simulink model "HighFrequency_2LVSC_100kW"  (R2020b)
settings: Solver=ode45  StartTime=0.0  StopTime=360  RelTol=1e-4  EnableMultiTasking=on
undefined symbols (not defined in the file): A, A_extheat, A_mp, AceH, AceL, ad0H, ad0L, ad1H, ad1L, ad2H, ad2L, AfH, AfL, at0H, at0L, at1H, at1L, at2H, at2L, C_V_ref, Cha1, CjcD, CjcT, Converters, Cp_Cu, Cp_wall, filter, FILTER_INT, fs, Grid_V, IGBT_len, IGBT_wid, Iq_init, J, k_box, k_mp, k_tp, kI_speed, kP_speed, L_equi, L_f1, Len_mp, Ls, nSpp, omega_m_init, omega_s, p, phi_pm, R1_cauer, R1D_bp, R2_cauer, R_f1, R_jc1, R_jc2, R_jc3, R_jc4, R_wall, Radius, RceH, RceL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
libraries: simulink x5, powerlib_meascontrol x2, pid_lib x2, cstblocks x1
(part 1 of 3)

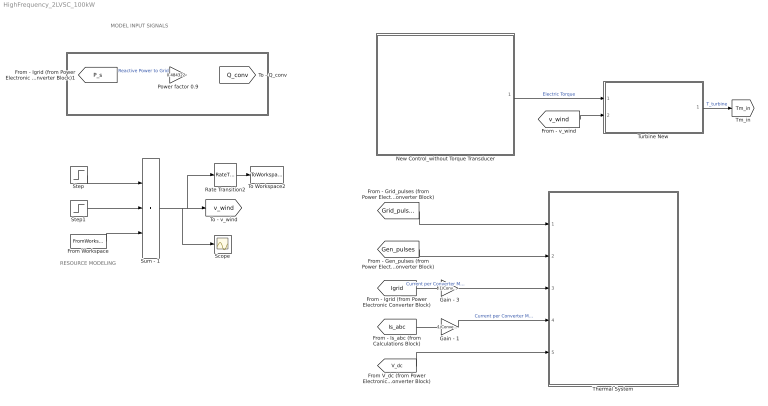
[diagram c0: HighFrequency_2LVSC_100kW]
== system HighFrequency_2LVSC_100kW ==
  note: RESOURCE MODELING
  note: MODEL INPUT SIGNALS
  "    " : Subsystem
  From Workspace : FromWorkspace  VariableName=vel_series  SampleTime=0.25
  Gain - 1 : Gain  Gain=1/Converters
  Gain - 3 : Gain  Gain=-1/Converters
  New Control_without Torque Transducer : Subsystem
  Power factor 0.9 : Gain  Gain=0.484322
  Rate Transition2 : RateTransition  OutPortSampleTime=1
  Scope : Scope
  Step : Step  Time=10  Before=0.52  After=v_tide  SampleTime=0
  Step1 : Step  Time=60  After=-v_tide  SampleTime=0
  Sum - 1 : Sum  Inputs=+++  InputSameDT=on  SaturateOnIntegerOverflow=on
  Thermal System : Subsystem
  To Workspace2 : ToWorkspace  VariableName=v_tide_simulink  SaveFormat=Structure With Time  SampleTime=-1
  Turbine New : Subsystem
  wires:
  New Control_without Torque Transducer/1(Torque_e) -> Turbine New/1(Electric Torque)  "Electric Torque"
  [P_s] -> Power factor 0.9/1  "Reactive Power to Grid"
  [v_wind] -> Turbine New/2(Tide Speed)
  Power factor 0.9/1 -> [Q_conv]
  Turbine New/1(T_load) -> [Tm_in]  "T_turbine"
  Step/1 -> Sum - 1/1
  [Is_abc] -> Gain - 1/1
  [V_dc] -> Thermal System/5(V_dc)
  Gain - 1/1 -> Thermal System/4(I_abc)  "Current per Converter Module"
  [Igrid] -> Gain - 3/1  "Current per Converter Module"
  [Gen_pulses] -> Thermal System/2(Gen_D)
  [Grid_pulses] -> Thermal System/1(Grid_D)
  Gain - 3/1 -> Thermal System/3(Igrid)
  Step1/1 -> Sum - 1/2
  From Workspace/1 -> Sum - 1/3
  Rate Transition2/1 -> To Workspace2/1
  Sum - 1/1 -> Scope/1, Rate Transition2/1, [v_wind]

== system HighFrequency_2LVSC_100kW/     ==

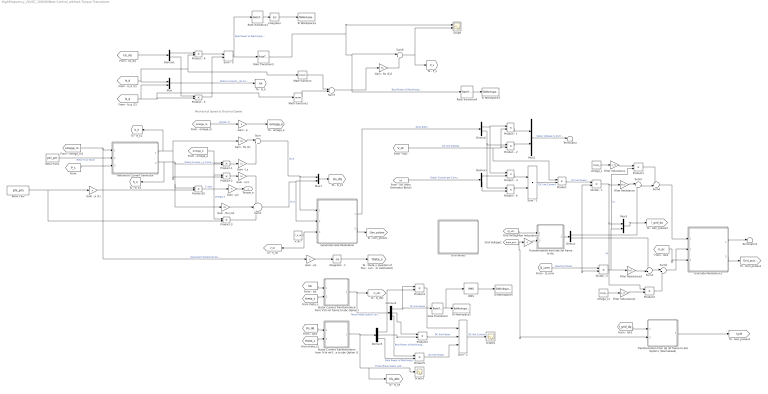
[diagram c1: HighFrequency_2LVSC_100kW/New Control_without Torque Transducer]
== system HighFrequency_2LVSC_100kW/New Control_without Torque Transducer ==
  note: Mechanical Speed to Electrical Speed
  Demux{,1..3} (4 alike) : Demux  Outputs=2
  Demux4 : Demux  Outputs=3
  Demux5 : Demux  Outputs=3
  Divide - 1 : Product  Inputs=*/
  Divide - 2 : Product  Inputs=*/
  Filter Inductance : Gain  Gain=L_f1
  Filter Inductance1 : Gain  Gain=L_f1
  Filter Inductance2 : Gain  Gain=-1
  Filter Resistance : Gain  Gain=R_f1
  "Filter Resistance2 " : Gain  Gain=R_f1
  Gain - Ls : Gain  Gain=Ls
  Gain - Ls1 : Gain  Gain=Ls
  Gain - Rs (1) : Gain  Gain=Rs
  Gain - Rs (1)1 : Gain  Gain=Rs
  Gain - Rs (1)2 : Gain  Gain=Rs
  Gain - p : Gain  Gain=p
  Gain - p (1) : Gain  Gain=p
  Gain - p1 : Gain  Gain=p
  Gain - p2 : Gain
  Generator-Side Modulation : Subsystem
  Grid Values : Subsystem
  Grid-Side Modulation1 : Subsystem
  Integrator : Integrator
  Integrator - 1 : Integrator  InitialCondition=theta_init
  Math Function : Math  Operator=square  SignedPower=on
  Math Function1 : Math  Operator=square  SignedPower=on
  Mux{,1..3} (4 alike) : Mux  Inputs=2
  Product{,1..5} (6 alike) : Product
  Product - {1..3,6} (4 alike) : Product
  Product - 4 : Product  InputSameDT=on  RndMeth=Zero  SaturateOnIntegerOverflow=on
  Product - 5 : Product  InputSameDT=on  RndMeth=Zero  SaturateOnIntegerOverflow=on
  Product-1 : Product  InputSameDT=on  RndMeth=Zero  SaturateOnIntegerOverflow=on
  Product-2 : Product  InputSameDT=on  RndMeth=Zero  SaturateOnIntegerOverflow=on
  Product-3 : Product  InputSameDT=on  RndMeth=Zero  SaturateOnIntegerOverflow=on
  Product10 : Product  InputSameDT=on  RndMeth=Zero  SaturateOnIntegerOverflow=on
  RMS : powerlib_meascontrol/Measurements/RMS  TrueRMS=on  Freq=13.7  RMSInit=120  Ts=0
  Rate Transition1 : RateTransition  OutPortSampleTime=0.001
  Rate Transition2 : RateTransition  OutPortSampleTime=0.001
  Rate Transition3 : RateTransition  OutPortSampleTime=0.1
  Rate Transition4 : RateTransition  OutPortSampleTime=1
  Reference Current Generator : Subsystem
  Rotor Flux : Constant  Value=phi_pm
  Rotor Flux1 : Constant  Value=phi_pm
  Scope : Scope  NumInputPorts=2
  Scope1 : Scope
  Scope2 : Scope
  Stator Current Transformation from 'k'th ref frame to abc Option I : Subsystem
  Stator Current Transformation from 'k'th ref frame to abc Option I1 : Subsystem
  Sum : Sum  Inputs=|+-
  Sum - 1 : Sum
  Sum - 2 : Sum  Inputs=+++
  Sum - 3 : Sum  InputSameDT=on  SaturateOnIntegerOverflow=on
  Sum1 : Sum  Inputs=+|+|+
  Sum2 : Sum  Inputs=|++
  Sum3 : Sum  Inputs=++|
  Sum4 : Sum  Inputs=-+|
  Sum5 : Sum  Inputs=|++
  Sum6 : Sum  Inputs=|+-
  Sum7 : Sum  Inputs=|++
  Terminator : Terminator
  Terminator1 : Terminator
  To Workspace1 : ToWorkspace  VariableName=P_gen  SaveFormat=Structure With Time  SampleTime=-1
  To Workspace2 : ToWorkspace  VariableName=IsGen_a  SaveFormat=Structure With Time  SampleTime=-1
  To Workspace3 : ToWorkspace  VariableName=Power_Gen1  SaveFormat=Structure With Time  SampleTime=1
  To Workspace4 : ToWorkspace  VariableName=IsGen_arms  SaveFormat=Structure With Time  SampleTime=-1
  "Transformation from abc ref frame to dq " : Subsystem
  Transformation from dq ref frame to abc Option I (Normalised) : Subsystem
  V_dc* : Constant  Value=C_V_ref
  omega_s : Constant  Value=omega_s
  omega_s1 : Constant  Value=omega_s
  Torque_e : Outport  VectorParamsAs1DForOutWhenUnconnected=off
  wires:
  [omega_m] -> Gain - p/1  "omega_m"
  Gain - p/1 -> [omega_e]
  Rotor Flux/1 -> Product-3/2, Gain - p (1)/1
  Gain - p (1)/1 -> Product10/2
  Product10/1 -> Gain - p2/1  "T_elec"
  Mux/1 -> [Isk]  "Stator Currents - dq Components"
  Demux1/1 -> Product - 4/1
  Demux1/2 -> Product - 5/1
  Product - 4/1 -> Sum - 3/1
  Product - 5/1 -> Sum - 3/2
  Sum - 3/1 -> Rate Transition1/1, Rate Transition3/1  "Real Power of Machine(pu)"
  [Is_d] -> Product - 4/2, Math Function/1, Mux/1
  [Is_q] -> Mux/2, Math Function1/1, Product - 5/2
  [Us_dq] -> Demux1/1
  Rotor Flux1/1 -> Reference Current Generator/2(Rotor Flux)  "Rotor Flux Value"
  [omega_m] -> Gain - p1/1, Reference Current Generator/1(omega_m)  "Generator Rotational Speed"
  Product-1/1 -> Gain - Ls/1
  [omega_e] -> Product-3/1, Product-2/1, Product-1/1  "omega_e"
  Reference Current Generator/2(I_q ref) -> [Is_q], Product-1/2, Gain - Rs (1)1/1, Product10/1  "Stator Current - q Component"
  Gain - Rs (1)/1 -> Sum/1
  Gain - Ls/1 -> Sum/2
  Sum/1 -> Generator-Side Modulation/1(Vd), Mux1/1  "Us_d"
  Reference Current Generator/1(I_d ref) -> [Is_d], Product-2/2, Gain - Rs (1)/1
  Product-2/1 -> Gain - Ls1/1
  Gain - Rs (1)1/1 -> Sum1/2
  Gain - Ls1/1 -> Sum1/1
  Product-3/1 -> Sum1/3
  Sum1/1 -> Generator-Side Modulation/2(Vq), Mux1/2  "Us_q"
  Mux1/1 -> [Us_dq]
  V_dc*/1 -> [V_dc], Generator-Side Modulation/3(Vdc)
  Generator-Side Modulation/2(Dabc) -> [Gen_pulses]
  Gain - p1/1 -> Integrator - 1/1
  Integrator - 1/1 -> [theta_s]
  [Isk] -> Stator Current Transformation from 'k'th ref frame to abc Option I/1("Is_{k}")
  [theta_s] -> Stator Current Transformation from 'k'th ref frame to abc Option I/2(theta_(s))
  Generator-Side Modulation/1(Ddq) -> Demux2/1  "Duty Ratio"
  Demux2/1 -> Product - 3/1, Product - 1/1
  [V_dc] -> Product/1, Product - 2/2, Product - 1/2  "DC link Voltage"
  Product - 1/1 -> Mux2/1
  Product - 2/1 -> Mux2/2
  Mux2/1 -> Terminator/1  "Stator Voltage in dq frame"
  Demux2/2 -> Product - 6/1, Product - 2/1
  [Isk] -> Demux3/1  "Stator Current per Converter Module"
  Demux3/1 -> Product - 3/2
  Demux3/2 -> Product - 6/2
  Product - 3/1 -> Sum - 1/1
  Product - 6/1 -> Sum - 1/2
  Sum - 1/1 -> Product/2  "DC link Current"
  Product/1 -> Divide - 1/1  "DC-link Power"
  [Vg_abc] -> "Transformation from abc ref frame to dq "/1(D_abc)
  [theta_grid] -> Transformation from dq ref frame to abc Option I (Normalised)/2(theta), Filter Inductance2/1
  "Transformation from abc ref frame to dq "/1(D_dq) -> Demux/1
  Demux/1 -> Sum2/2, Divide - 1/2, Divide - 2/2
  Divide - 1/1 -> Mux3/1, Product2/1, Filter Resistance/1  "Id"
  [Q_conv] -> Divide - 2/1  "Reactive Power"
  Divide - 2/1 -> "Filter Resistance2 "/1, Mux3/2, Product1/2  "Iq"
  omega_s/1 -> Filter Inductance/1
  Filter Resistance/1 -> Sum2/1
  "Filter Resistance2 "/1 -> Sum3/2
  Demux/2 -> Sum3/1
  Sum2/1 -> Sum4/2
  Filter Inductance/1 -> Product1/1
  Product1/1 -> Sum4/1
  omega_s1/1 -> Filter Inductance1/1
  Filter Inductance1/1 -> Product2/2
  Sum3/1 -> Sum5/1
  Product2/1 -> Sum5/2
  Sum4/1 -> Grid-Side Modulation1/1(Vd)
  Sum5/1 -> Grid-Side Modulation1/2(Vq)
  [V_dc] -> Grid-Side Modulation1/3(Vdc)
  Grid-Side Modulation1/2(Dabc) -> [Grid_pulses]
  Grid-Side Modulation1/1(Ddq) -> Terminator1/1
  Mux3/1 -> [I_grid_dq]
  [I_grid_dq] -> Transformation from dq ref frame to abc Option I (Normalised)/1(D_dq)
  Transformation from dq ref frame to abc Option I (Normalised)/1(D_abc) -> [Igrid]
  Filter Inductance2/1 -> "Transformation from abc ref frame to dq "/2(theta_(s))
  [Us_dq] -> Stator Current Transformation from 'k'th ref frame to abc Option I1/1("Is_{k}")
  [theta_s] -> Stator Current Transformation from 'k'th ref frame to abc Option I1/2(theta_(s))
  Rate Transition1/1 -> Integrator/1
  Integrator/1 -> To Workspace1/1
  [P_s] -> Reference Current Generator/3("P_in ")
  Gain - p2/1 -> Torque_e/1
  Demux4/2 -> Product3/1
  Demux4/1 -> Product4/1, Rate Transition2/1
  Stator Current Transformation from 'k'th ref frame to abc Option I/1("Is_{abc}") -> Demux4/1, [Is_abc]  "Three Phase Stator Currents"
  Stator Current Transformation from 'k'th ref frame to abc Option I1/1("Is_{abc}") -> [Us_abc], Scope1/1, Demux5/1  "Three Phase Stator voltage"
  Demux5/2 -> Product3/2
  Demux5/1 -> Product4/2
  Demux4/3 -> Product5/1  "Real Power of Machine(pu)"
  Demux5/3 -> Product5/2  "Real Power of Machine(pu)"
  Product3/1 -> Sum - 2/2  "DC-link Power"
  Product4/1 -> Sum - 2/1  "DC-link Power"
  Product5/1 -> Sum - 2/3  "DC-link Power"
  Sum - 2/1 -> Scope2/1  "DC link Current"
  Gain - Rs (1)2/1 -> Sum6/2
  Math Function/1 -> Sum7/1
  Math Function1/1 -> Sum7/2
  Sum7/1 -> Gain - Rs (1)2/1
  Sum6/1 -> [P_s], Scope/2
  RMS/1 -> To Workspace4/1
  Rate Transition2/1 -> RMS/1, To Workspace2/1
  Rate Transition4/1 -> To Workspace3/1
  Rate Transition3/1 -> Rate Transition4/1, Sum6/1, Scope/1  "Real Power of Machine(pu)"

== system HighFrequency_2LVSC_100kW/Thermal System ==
  Grid_D : Inport
  Gen_D : Inport  Port=2
  Igrid : Inport  Port=3
  I_abc : Inport  Port=4
  V_dc : Inport  Port=5
  Select Leg (Select Converter Leg for Thermal Model) : Constant
  Thermal Model - Generator Side : Subsystem
  Thermal Model - Grid Side : Subsystem  Commented=on
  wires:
  Igrid/1 -> Thermal Model - Grid Side/2(I_abc)
  Grid_D/1 -> Thermal Model - Grid Side/1(D_abc)
  V_dc/1 -> Thermal Model - Grid Side/3(V_dc), Thermal Model - Generator Side/3(V_dc)
  I_abc/1 -> Thermal Model - Generator Side/2(I_abc)
  Gen_D/1 -> Thermal Model - Generator Side/1(D_abc)
  Select Leg (Select Converter Leg for Thermal Model)/1 -> [Phase]

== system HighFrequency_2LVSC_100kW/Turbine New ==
  Electric Torque : Inport
  Tide Speed : Inport  Port=2
  Mechanical System : Subsystem
  Product - 1 : Product  Commented=on  RndMeth=Zero
  Rate Transition1 : RateTransition  OutPortSampleTime=Ts_out/5
  Rate Transition2 : RateTransition  OutPortSampleTime=Ts_out/5
  Rotor Model : Subsystem
  Scope : Scope
  To Workspace1 : ToWorkspace  VariableName=Gen_loadT  SaveFormat=Structure With Time  SampleTime=-1
  To Workspace2 : ToWorkspace  VariableName=v_tide_struct  SaveFormat=Structure With Time  SampleTime=-1
  T_load : Outport  VectorParamsAs1DForOutWhenUnconnected=off
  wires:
  Mechanical System/1(omega_m) -> Rotor Model/1(omega_m), Product - 1/2, [omega_m]  "Generator Rotational Speed"
  Electric Torque/1 -> Mechanical System/1(Electric Torque)  "T_elec"
  Rate Transition1/1 -> To Workspace1/1
  Tide Speed/1 -> Rate Transition2/1, Rotor Model/2(Wind Speed)
  Rate Transition2/1 -> To Workspace2/1
  Rotor Model/1(T_load) -> Product - 1/1, Rate Transition1/1, T_load/1, Mechanical System/2(Load Torque)
  Product - 1/1 -> Scope/1

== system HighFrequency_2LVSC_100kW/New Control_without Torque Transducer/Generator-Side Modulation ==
  Vd : Inport
  Vq : Inport  Port=2
  Vdc : Inport  Port=3
  Divide - 1 : Product  Inputs=*/
  Duty Limits : Saturate
  Gain - 1 : Gain  Gain=2
  Mux2 : Mux  Inputs=2
  Third Harmonic Injection : Subsystem
  Transformation from abc ref frame to dq Option I (Normalised) : Subsystem
  Transformation from dq ref frame to abc Option I (Normalised) : Subsystem
  Ddq : Outport  VectorParamsAs1DForOutWhenUnconnected=off
  Dabc : Outport  Port=2  VectorParamsAs1DForOutWhenUnconnected=off
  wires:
  Third Harmonic Injection/1(V_out) -> Duty Limits/1
  Duty Limits/1 -> Gain - 1/1, Transformation from abc ref frame to dq Option I (Normalised)/1(D_abc)
  Gain - 1/1 -> Dabc/1
  Divide - 1/1 -> Transformation from dq ref frame to abc Option I (Normalised)/1(D_dq)  "Duty Ratio"
  Transformation from abc ref frame to dq Option I (Normalised)/1(D_dq) -> Ddq/1
  [theta_s] -> Transformation from dq ref frame to abc Option I (Normalised)/2(theta), Transformation from abc ref frame to dq Option I (Normalised)/2(theta_(s))
  Vdc/1 -> Divide - 1/2
  Mux2/1 -> Divide - 1/1
  Vd/1 -> Mux2/1
  Vq/1 -> Mux2/2
  Transformation from dq ref frame to abc Option I (Normalised)/1(D_abc) -> Third Harmonic Injection/1(V_in)

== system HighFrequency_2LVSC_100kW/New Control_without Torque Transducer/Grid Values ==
  Create 3 Phase Voltage Signal (in lieu of Grid Model) : Subsystem
  Grid Voltage (from Initialisation file) : Constant  Value=Grid_V
  Mux3 : Mux  Inputs=3
  Voltage Angle in dq : Subsystem
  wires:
  Mux3/1 -> Voltage Angle in dq/1(Three Phase Voltages), [Vg_abc], [Usabc]
  Create 3 Phase Voltage Signal (in lieu of Grid Model)/3(Phase C Voltage) -> Mux3/3
  Create 3 Phase Voltage Signal (in lieu of Grid Model)/1(Phase A Voltage) -> Mux3/1
  Grid Voltage (from Initialisation file)/1 -> Create 3 Phase Voltage Signal (in lieu of Grid Model)/1(Grid Voltage)
  Create 3 Phase Voltage Signal (in lieu of Grid Model)/2(Phase B Voltage) -> Mux3/2
  Voltage Angle in dq/1(angle) -> [theta_grid]

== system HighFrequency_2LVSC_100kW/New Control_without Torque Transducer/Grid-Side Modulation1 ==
  Vd : Inport
  Vq : Inport  Port=2
  Vdc : Inport  Port=3
  Divide - 1 : Product  Inputs=*/
  Duty Limits : Saturate
  Gain - 1 : Gain  Gain=2
  Mux2 : Mux  Inputs=2
  Third Harmonic Injection : Subsystem
  Transformation from abc ref frame to dq Option I (Normalised) : Subsystem
  Transformation from dq ref frame to abc Option I (Normalised) : Subsystem
  Ddq : Outport  VectorParamsAs1DForOutWhenUnconnected=off
  Dabc : Outport  Port=2  VectorParamsAs1DForOutWhenUnconnected=off
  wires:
  Third Harmonic Injection/1(V_out) -> Duty Limits/1
  Duty Limits/1 -> Gain - 1/1, Transformation from abc ref frame to dq Option I (Normalised)/1(D_abc)
  Gain - 1/1 -> Dabc/1
  Divide - 1/1 -> Transformation from dq ref frame to abc Option I (Normalised)/1(D_dq)  "Duty Ratio"
  Transformation from abc ref frame to dq Option I (Normalised)/1(D_dq) -> Ddq/1
  [theta_grid] -> Transformation from dq ref frame to abc Option I (Normalised)/2(theta), Transformation from abc ref frame to dq Option I (Normalised)/2(theta_(s))
  Vdc/1 -> Divide - 1/2
  Mux2/1 -> Divide - 1/1
  Vd/1 -> Mux2/1
  Vq/1 -> Mux2/2
  Transformation from dq ref frame to abc Option I (Normalised)/1(D_abc) -> Third Harmonic Injection/1(V_in)

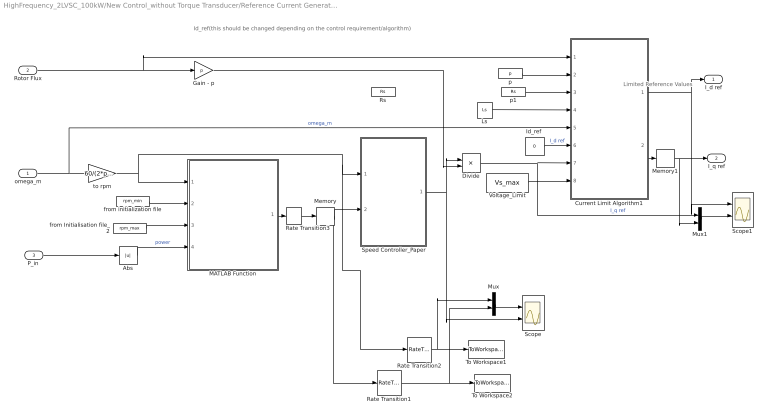
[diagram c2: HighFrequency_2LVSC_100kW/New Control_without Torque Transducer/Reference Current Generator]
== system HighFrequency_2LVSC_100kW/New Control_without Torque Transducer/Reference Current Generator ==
  note: Id_ref(this should be changed depending on the control requirement/algorithm)
  note: Limited Reference Values
  omega_m : Inport
  Rotor Flux : Inport  Port=2
  "P_in " : Inport  Port=3
  Abs : Abs  ZeroCross=off
  Current Limit Algorithm1 : MATLAB Function  TreatAsAtomicUnit=on
  Divide : Product  Inputs=*/
  Gain - p : Gain  Gain=p
  "Id_ref " : Constant  Value=0
  Ls : Constant  Value=Ls
  MATLAB Function : MATLAB Function  TreatAsAtomicUnit=on
  Memory : Memory  InitialCondition=omega_m_init*60/2/pi  InheritSampleTime=on
  Memory1 : Memory  InitialCondition=Iq_init  InheritSampleTime=on
  Mux : Mux  Inputs=2
  Mux1 : Mux  Inputs=2
  Rate Transition1 : RateTransition  OutPortSampleTime=1
  Rate Transition2 : RateTransition  OutPortSampleTime=1
  Rate Transition3 : RateTransition  OutPortSampleTime=0.1
  Rs : Constant  Commented=on  Value=Rs
  Scope : Scope  NumInputPorts=2
  Scope1 : Scope  NumInputPorts=2
  Speed Controller_Paper : Subsystem  mask(Speed controller){SwK=Speed regulation, fn=rpm_rated*p/60, ramp=[-1,1]*2, kp=kP_speed, ki=kI_speed, kd=0, fc=100*100, ctrl_sat=[-1000, 1000]*8.7*1.5*50, p=p, nf=phi_pm, Tsc=1e-5}
      mask prompts: SwK "Regulation type"; fn "Machine nominal frequency (Hz)"; ramp "Speed reference ramp  (rpm/s) [deceleration,acceleration]"; kp "Proportional Gain"; ki "Integral Gain"; kd "Derivative Gain"; fc "Speed measurement - low-pass filter cutoff frequency (Hz)"; ctrl_sat "Controller output torque saturation (N.m) [negative,positive]"; p "Motor pairs of poles"; nf "Machine nominal flux (Wb)"; Tsc "Controller sampling time (s)"
      mask help: This block implements a PI speed regulator.
      mask init:
      | bs=2*30*fn/p;
      | [X1,X1m,X2,X2m,X3,X4,Y1,Y1m,Y2,Y2m,Y3,Y4,color1,color2]=spsdrivelogo;
      | if SwK == 1
      |     set_param(gcb,'MaskVisibilities',{'on','on','on','on','on','on','on','on','on','on','on'})
      | else
      |     set_param(gcb,'MaskVisibilities',{'on','on','off','off','off','off','off','on','on','on','on'})
      | end
  To Workspace1 : ToWorkspace  VariableName=N_gen_plot  SaveFormat=Structure With Time  SampleTime=1
  To Workspace2 : ToWorkspace  VariableName=N_gen_ref  SaveFormat=Structure With Time  SampleTime=1
  Voltage_Limit : Constant  Value=Vs_max
  from Initialisation file_2 : Constant  Value=rpm_max
  from initialization file : Constant  Value=rpm_min
  p : Constant  Value=p
  p1 : Constant  Value=Rs
  to rpm : Gain  Gain=60/(2*pi)
  I_d ref : Outport  VectorParamsAs1DForOutWhenUnconnected=off
  I_q ref : Outport  Port=2  VectorParamsAs1DForOutWhenUnconnected=off
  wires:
  omega_m/1 -> Current Limit Algorithm1/5(omega_m), to rpm/1  "omega_m"
  Rotor Flux/1 -> Current Limit Algorithm1/1(rot_f), Gain - p/1
  "P_in "/1 -> Abs/1
  Current Limit Algorithm1/1(isdref) -> Scope1/1, I_d ref/1
  "Id_ref "/1 -> Current Limit Algorithm1/6(isd)  "I_d ref"
  Current Limit Algorithm1/2(isqref) -> Memory1/1
  Divide/1 -> Mux1/1, Current Limit Algorithm1/7(isq)  "I_q ref"
  Memory1/1 -> Mux1/2, I_q ref/1
  Mux/1 -> Scope/1
  Speed Controller_Paper/1(Torque*) -> Divide/1, Scope/2
  Gain - p/1 -> Divide/2
  from initialization file/1 -> MATLAB Function/2(Nrpmmin)
  from Initialisation file_2/1 -> MATLAB Function/3(Nrpmmax)
  to rpm/1 -> MATLAB Function/1(Nrpm), Speed Controller_Paper/1(N), Rate Transition2/1
  Memory/1 -> Rate Transition1/1, Speed Controller_Paper/2(N*)
  Rate Transition2/1 -> Mux/1, To Workspace1/1
  Rate Transition1/1 -> Mux/2, To Workspace2/1
  Abs/1 -> MATLAB Function/4(P_in)  "power"
  Rate Transition3/1 -> Memory/1
  MATLAB Function/1(N_ref) -> Rate Transition3/1
  Voltage_Limit/1 -> Current Limit Algorithm1/8(Vs_max)
  Ls/1 -> Current Limit Algorithm1/4(Ls)
  p/1 -> Current Limit Algorithm1/2(p)
  p1/1 -> Current Limit Algorithm1/3(Rs)
  Mux1/1 -> Scope1/2

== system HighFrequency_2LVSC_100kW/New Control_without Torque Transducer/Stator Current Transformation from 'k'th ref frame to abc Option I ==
  "Is_{k}" : Inport
  theta_(s) : Inport  Port=2
  Clarke Transform : Subsystem
  Demux : Demux  Outputs=2
  Gain : Gain  Gain=-1
  Mux : Mux  Inputs=3
  "Park Transform " : Subsystem
  "Is_{abc}" : Outport  VectorParamsAs1DForOutWhenUnconnected=off
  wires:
  Clarke Transform/1(out_1) -> Mux/1
  Clarke Transform/3(out_3) -> Mux/3
  Clarke Transform/2(out_2) -> Mux/2
  "Park Transform "/2(out_2) -> Clarke Transform/2(in_2)
  "Park Transform "/1(out_1) -> Clarke Transform/1(in_1)
  Gain/1 -> "Park Transform "/3(in_3)
  "Is_{k}"/1 -> Demux/1
  Mux/1 -> "Is_{abc}"/1
  Demux/1 -> "Park Transform "/1(in_1)
  Demux/2 -> "Park Transform "/2(in_2)
  theta_(s)/1 -> Gain/1

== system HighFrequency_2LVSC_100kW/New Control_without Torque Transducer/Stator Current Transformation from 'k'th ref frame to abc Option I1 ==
  "Is_{k}" : Inport
  theta_(s) : Inport  Port=2
  Clarke Transform : Subsystem
  Demux : Demux  Outputs=2
  Gain : Gain  Gain=-1
  Mux : Mux  Inputs=3
  "Park Transform " : Subsystem
  "Is_{abc}" : Outport  VectorParamsAs1DForOutWhenUnconnected=off
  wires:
  theta_(s)/1 -> Gain/1
  Demux/2 -> "Park Transform "/2(in_2)
  Demux/1 -> "Park Transform "/1(in_1)
  Mux/1 -> "Is_{abc}"/1
  "Is_{k}"/1 -> Demux/1
  Gain/1 -> "Park Transform "/3(in_3)
  "Park Transform "/1(out_1) -> Clarke Transform/1(in_1)
  "Park Transform "/2(out_2) -> Clarke Transform/2(in_2)
  Clarke Transform/2(out_2) -> Mux/2
  Clarke Transform/3(out_3) -> Mux/3
  Clarke Transform/1(out_1) -> Mux/1

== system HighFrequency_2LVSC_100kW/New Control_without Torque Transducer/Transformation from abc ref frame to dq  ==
  D_abc : Inport
  theta_(s) : Inport  Port=2
  Clarke Transform : Subsystem
  Demux : Demux  Outputs=3
  Mux1 : Mux  Inputs=2
  Parks Transform : Subsystem
  D_dq : Outport  VectorParamsAs1DForOutWhenUnconnected=off
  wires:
  Parks Transform/1(out_1) -> Mux1/1
  Parks Transform/2(out_2) -> Mux1/2
  D_abc/1 -> Demux/1
  Mux1/1 -> D_dq/1
  Demux/1 -> Clarke Transform/1(in_1)
  Demux/2 -> Clarke Transform/2(in_2)
  Demux/3 -> Clarke Transform/3(in_3)
  Clarke Transform/1(out_1) -> Parks Transform/1(in_1)
  Clarke Transform/2(out_2) -> Parks Transform/2(in_2)
  theta_(s)/1 -> Parks Transform/3(in_3)

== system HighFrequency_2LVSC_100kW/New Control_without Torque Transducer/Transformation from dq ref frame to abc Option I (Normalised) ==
  D_dq : Inport
  theta : Inport  Port=2
  Clarke Transform : Subsystem
  Demux : Demux  Outputs=2
  Gain : Gain  Gain=-1
  Mux1 : Mux  Inputs=3
  Parks Transform : Subsystem
  D_abc : Outport  VectorParamsAs1DForOutWhenUnconnected=off
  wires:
  Parks Transform/2(out_2) -> Clarke Transform/2(in_2)
  Parks Transform/1(out_1) -> Clarke Transform/1(in_1)
  Gain/1 -> Parks Transform/3(in_3)
  D_dq/1 -> Demux/1
  Mux1/1 -> D_abc/1
  Demux/1 -> Parks Transform/1(in_1)
  Demux/2 -> Parks Transform/2(in_2)
  theta/1 -> Gain/1
  Clarke Transform/3(out_3) -> Mux1/3
  Clarke Transform/2(out_2) -> Mux1/2
  Clarke Transform/1(out_1) -> Mux1/1

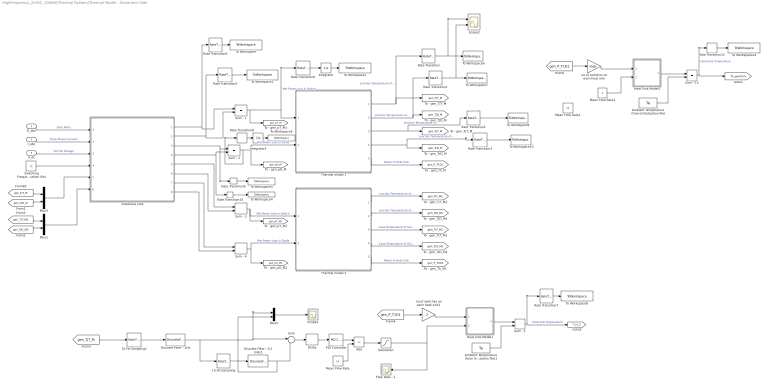
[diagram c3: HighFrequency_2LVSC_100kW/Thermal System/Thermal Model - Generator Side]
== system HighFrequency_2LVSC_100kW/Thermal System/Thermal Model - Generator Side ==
  D_abc : Inport
  I_abc : Inport  Port=2
  V_dc : Inport  Port=3
  10 Hz Sampling : RateTransition  Commented=on  InitialCondition=60  OutPortSampleTime=1e-1
  10 Hz Sampling1 : RateTransition  Commented=on  InitialCondition=60  OutPortSampleTime=1e-3
  Add : Sum  Commented=on  Inputs=-+
  Ambient Temperature (from Initialisation file) : Constant  Value=Ta
  Ambient Temperature (from Initialisation file)1 : Constant  Commented=on  Value=Ta
  Delay : Delay  Commented=on  DelayLength=1  InitialCondition=0  SampleTime=1e-3
  Discrete Filter - 0.1 mHz1 : DiscreteFilter  Commented=on  Numerator=[1 1]  Denominator=[1]  InitialStates=1
  Discrete Filter - 1Hz : DiscreteFilter  Commented=on  Numerator=[1 1]  Denominator=FILTER_INT  InitialStates=filter
  Flow Rate - 1 : Scope
  Heat Sink Model1 : Subsystem  Commented=on
  Heat Sink Model2 : Subsystem
  Instanous Loss : Subsystem
  Integrator : Integrator
  Integrator1 : Integrator
  Mean Flow Rate : Constant  Commented=on  Value=15
  Mean Flow Rate1 : Constant  Commented=on  Value=15
  Mean Flow Rate2 : Constant
  Mux1 : Mux  Inputs=2
  Mux2 : Mux  Commented=on  Inputs=2
  Mux3 : Mux  Inputs=2
  PID Controller : pid_lib/PID Controller  Commented=on  Controller=P  Form=Parallel  TimeDomain=Continuous-time  UseExternalTs=off  SampleTime=-1  IntegratorMethod=Forward Euler  FilterMethod=Forward Euler  ControllerParametersSource=internal  P=25  I=0.005  D=0  UseFilter=on  N=100  TunerSelectOption=Transfer Function Based (PID Tuner App)  InitialConditionSource=internal  InitialConditionForIntegrator=15  InitialConditionForFilter=0  DifferentiatorICPrevScaledInput=0  ExternalReset=none  TrackingMode=off  Kt=1  LimitOutput=off  SatLimitsSource=internal  UpperSaturationLimit=inf  LowerSaturationLimit=-inf  LinearizeAsGain=on  AntiWindupMode=none  Kb=1  POutMin=[]  POutMax=[]  IOutMin=[]  IOutMax=[]  DOutMin=[]  DOutMax=[]  NOutMin=[]  NOutMax=[]  SumOutMin=[]  SumOutMax=[]  SaturationOutMin=[]  SaturationOutMax=[]  PParamMin=[]  PParamMax=[]  IParamMin=[]  IParamMax=[]  DParamMin=[]  DParamMax=[]  NParamMin=[]  NParamMax=[]  KbParamMin=[]  KbParamMax=[]  KtParamMin=[]  KtParamMax=[]  KbOutMin=[]  KbOutMax=[]  KtOutMin=[]  KtOutMax=[]  IntegratorOutMin=[]  IntegratorOutMax=[]  FilterOutMin=[]  FilterOutMax=[]  SumI1OutMin=[]  SumI1OutMax=[]  SumI2OutMin=[]  SumI2OutMax=[]  SumI3OutMin=[]  SumI3OutMax=[]  SumI4OutMin=[]  SumI4OutMax=[]  SumDOutMin=[]  SumDOutMax=[]  DifferentiatorOutMin=[]  DifferentiatorOutMax=[]  FilterDiffOutCoefMin=[]  FilterDiffOutCoefMax=[]  ReciprocalOutMin=[]  ReciprocalOutMax=[]  SumDenOutMin=[]  SumDenOutMax=[]  SumNumOutMin=[]  SumNumOutMax=[]  DivideOutMin=[]  DivideOutMax=[]  UdiffTsProdOutMin=[]  UdiffTsProdOutMax=[]  NTsProdOutMin=[]  NTsProdOutMax=[]  UintegralTsProdOutMin=[]  UintegralTsProdOutMax=[]  UngainTsProdOutMin=[]  UngainTsProdOutMax=[]  IntegratorContinuousStateAttributes=''  IntegratorStateMustResolveToSignalObject=off  IntegratorRTWStateStorageClass=Auto  FilterContinuousStateAttributes=''  FilterStateMustResolveToSignalObject=off  FilterRTWStateStorageClass=Auto  ParallelPVariant=InternalParameters  IdealPVariant=Disabled  IVariant=Disabled  DVariant=Disabled  IntegratorVariant=Disabled  SatVariant=Disabled  AWVariant=Disabled  PCopyVariant=Disabled  TRVariant=Disabled  FdbkBlocksVariant=Forward  IdealPFdbkVariant=Disabled  SatFdbkVariant=Disabled  DerivativeFilterVariant=Disabled  NVariant=Disabled  NCopyVariant=Disabled_SignalSpec  FilterICVariant=Disabled  IntegratorICVariant=Disabled  ExternalResetVariant=Disabled  TRSumVariant=Passthrough  SumFdbkVariant=Disabled  SumVariant=Passthrough_P  TsampFilterVariant=InternalTs  TsampNgainVariant=Passthrough  TsampIntegralVariant=Disabled_SignalSpec  ExternalSaturationOutDataTypeStr=Inherit: Same as second input
  Rate Transition{,1..3,6,8} (6 alike) : RateTransition  OutPortSampleTime=Ts_out
  Rate Transition10 : RateTransition  OutPortSampleTime=0.001
  Rate Transition12 : RateTransition  OutPortSampleTime=Ts_out_lf
  Rate Transition4 : RateTransition  Commented=on  OutPortSampleTime=Ts_out
  Rate Transition5 : RateTransition  Commented=on  OutPortSampleTime=Ts_out
  Rate Transition7 : RateTransition  Commented=on  OutPortSampleTime=0.001
  Rate Transition9 : RateTransition  OutPortSampleTime=0.001
  Saturation : Saturate  Commented=on  UpperLimit=15  LowerLimit=0
  Scope2 : Scope  NumInputPorts=2
  Scope3 : Scope
  Sum : Sum  Commented=on  Inputs=|-+
  Sum - {1..4,15} (5 alike) : Sum
  Sum - 5 : Sum  Commented=on
  Switching Frequency (from Initialisation file) : Constant  Value=fs
  Thermal model 1 : Subsystem
  Thermal model 2 : Subsystem  Commented=on
  To Workspace : ToWorkspace  VariableName=gen_P_cond_T1  SaveFormat=Structure With Time  SampleTime=-1
  To Workspace1 : ToWorkspace  VariableName=gen_P_sw_T1  SaveFormat=Structure With Time  SampleTime=-1
  To Workspace10 : ToWorkspace  VariableName=gen_T_cD1  SaveFormat=Structure With Time  SampleTime=-1
  To Workspace2 : ToWorkspace  VariableName=gen_P_netT1  SaveFormat=Structure With Time  SampleTime=-1
  To Workspace24 : ToWorkspace  VariableName=Th_Gen  SaveFormat=Structure With Time  SampleTime=-1
  To Workspace3 : ToWorkspace  VariableName=gen_P_cond_D1  SaveFormat=Structure With Time  SampleTime=-1
  To Workspace4 : ToWorkspace  VariableName=gen_P_sw_D1  SaveFormat=Structure With Time  SampleTime=-1
  To Workspace5 : ToWorkspace  VariableName=gen_P_netD1  SaveFormat=Structure With Time  SampleTime=-1
  To Workspace6 : ToWorkspace  VariableName=gen_T_jT1  SaveFormat=Structure With Time  SampleTime=-1
  To Workspace7 : ToWorkspace  VariableName=gen_T_jD1  SaveFormat=Structure With Time  SampleTime=-1
  To Workspace8 : ToWorkspace  VariableName=T_h_C  SaveFormat=Structure With Time  SampleTime=-1
  To Workspace9 : ToWorkspace  VariableName=gen_T_cT1  SaveFormat=Structure With Time  SampleTime=-1
  no.of switches on each heat sink : Gain  Gain=nSpp
  no.of switches on each heat sink1 : Gain  Commented=on  Gain=2
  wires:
  D_abc/1 -> Instanous Loss/1(D_abc)  "Duty Ratio"
  I_abc/1 -> Instanous Loss/2(I_abc)  "Three Phase Currents"
  V_dc/1 -> Instanous Loss/3(Vdc)  "DC link Voltage"
  Switching Frequency (from Initialisation file)/1 -> Instanous Loss/4(fs)
  Sum - 1/1 -> [gen_pT_M], Rate Transition6/1, Thermal model 1/1(ploss_T1)  "Net Power Loss in Switch"
  Instanous Loss/1(pconT1_Tj) -> Sum - 1/1, Rate Transition4/1
  Instanous Loss/2(pswT1_Tj) -> Sum - 1/2, Rate Transition5/1
  Instanous Loss/3(pconD1_Tj) -> Sum - 2/1, Rate Transition9/1
  Instanous Loss/4(pswD1_Tj) -> Rate Transition10/1, Sum - 2/2
  Sum - 2/1 -> [gen_pD_M], Thermal model 1/2(ploss_D1), Rate Transition8/1  "Net Power Loss in Diode"
  Thermal model 1/5(P_T1/D1) -> [gen_P_T1D1]  "Power to Heat Sink"
  [gen_TjT_M] -> Mux3/1
  [gen_TjD_M] -> Mux3/2
  Mux3/1 -> Instanous Loss/5(Tj_T1D1)
  [gen_TjT_M2] -> Mux1/1
  [gen_TjD_M2] -> Mux1/2
  Mux1/1 -> Instanous Loss/6(Tj_T2D2)
  Sum - 3/1 -> [gen_pT_M2], Thermal model 2/1(ploss_T2)  "Net Power Loss in Switch"
  Instanous Loss/5(pconT2_Tj) -> Sum - 3/1
  Instanous Loss/6(pswT2_Tj) -> Sum - 3/2
  Thermal model 2/1(TjT2) -> [gen_TjT_M2]  "Junction Temperature of Switch"
  Instanous Loss/7(pconD2_Tj) -> Sum - 4/1
  Instanous Loss/8(pswD2_Tj) -> Sum - 4/2
  Sum - 4/1 -> [gen_pD_M2], Thermal model 2/2(ploss_D1)  "Net Power Loss in Diode"
  Thermal model 2/2(TjD2) -> [gen_TjD_M2]  "Junction Temperature of Diode"
  Thermal model 2/3(TcT2) -> [gen_TcT_M2]  "Case Temperature of Switch"
  Thermal model 2/4(TcD2) -> [gen_TcD_M2]  "Case Temperature of Diode"
  Thermal model 2/5(P_T2/D2) -> [gen_P_T2D2]  "Power to Heat Sink"
  Thermal model 1/1(TjT1) -> Rate Transition/1, [gen_TjT_M]  "Junction Temperature of Switch"
  Thermal model 1/2(TjD1) -> Rate Transition1/1, [gen_TjD_M]  "Junction Temperature of Switch"
  Rate Transition/1 -> Scope2/1, To Workspace6/1
  Rate Transition1/1 -> Scope2/2, To Workspace7/1
  Thermal model 1/3(TcT1) -> Rate Transition2/1, [gen_TcT_M]  "Junction Temperature of Switch"
  Thermal model 1/4(TcD1) -> Rate Transition3/1, [gen_TcD_M]  "Junction Temperature of Switch"
  Rate Transition2/1 -> To Workspace9/1
  Rate Transition3/1 -> To Workspace10/1
  Rate Transition4/1 -> To Workspace/1
  Rate Transition5/1 -> To Workspace1/1
  Rate Transition6/1 -> Integrator/1
  Rate Transition9/1 -> To Workspace3/1
  Rate Transition10/1 -> To Workspace4/1
  Integrator/1 -> To Workspace2/1
  Rate Transition8/1 -> Integrator1/1
  Integrator1/1 -> To Workspace5/1
  Sum - 15/1 -> [Th_genConv], Rate Transition12/1  "Heat Sink Temperature"
  Heat Sink Model2/1(Tha1) -> Sum - 15/1
  Ambient Temperature (from Initialisation file)/1 -> Sum - 15/2
  [gen_P_T1D1] -> no.of switches on each heat sink/1
  Rate Transition12/1 -> To Workspace24/1
  10 Hz Sampling/1 -> Discrete Filter - 0.1 mHz1/1
  Heat Sink Model1/1(Tha1) -> Sum - 5/1
  Delay/1 -> PID Controller/1
  [gen_P_T1D1] -> no.of switches on each heat sink1/1
  10 Hz Sampling1/1 -> Discrete Filter - 1Hz/1
  Discrete Filter - 0.1 mHz1/1 -> Mux2/2, Sum/2
  Add/1 -> Saturation/1
  Discrete Filter - 1Hz/1 -> 10 Hz Sampling/1, Mux2/1, Sum/1
  Mux2/1 -> Scope3/1
  Sum/1 -> Delay/1
  [gen_TjT_M] -> 10 Hz Sampling1/1
  Saturation/1 -> Heat Sink Model1/2(Flow Rate), Flow Rate - 1/1
  Rate Transition7/1 -> To Workspace8/1
  Sum - 5/1 -> Rate Transition7/1, [T_h1_C]  "Heat Sink Temperature"
  PID Controller/1 -> Add/1
  Ambient Temperature (from Initialisation file)1/1 -> Sum - 5/2
  Mean Flow Rate/1 -> Add/2
  no.of switches on each heat sink/1 -> Heat Sink Model2/1(PT1/D1)
  no.of switches on each heat sink1/1 -> Heat Sink Model1/1(PT1/D1)
  Mean Flow Rate2/1 -> Heat Sink Model2/2(Flow Rate)

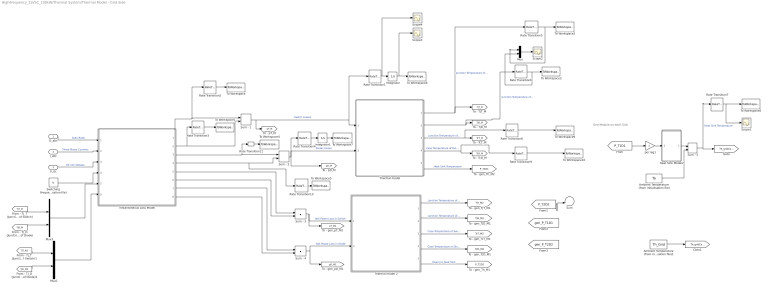
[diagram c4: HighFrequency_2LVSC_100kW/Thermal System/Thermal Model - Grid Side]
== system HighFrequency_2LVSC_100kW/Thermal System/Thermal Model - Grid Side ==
  note: One Module on each Sink
  D_abc : Inport
  I_abc : Inport  Port=2
  V_dc : Inport  Port=3
  Ambient Temperature (from Initialisation file) : Constant  Commented=on  Value=Ta
  Ambient Temperature (from Initialisation file)1 : Constant  Value=Th_Grid
  Heat Sink Model2 : Subsystem  Commented=on
  Instantaneous Loss Model : Subsystem
  Integrator : Integrator
  Integrator1 : Integrator
  Mux : Mux  Inputs=2
  Mux1 : Mux  Inputs=2
  Mux3 : Mux  Inputs=2
  Rate Transition{1..6,8..9,11} (9 alike) : RateTransition  OutPortSampleTime=Ts_out
  Rate Transition10 : RateTransition  Commented=on  OutPortSampleTime=Ts_out
  Rate Transition7 : RateTransition  Commented=on  OutPortSampleTime=Ts_out
  Scope{1..4} (4 alike) : Scope
  Sum : Sum  Commented=on  Inputs=|++
  Sum - {1..4} (4 alike) : Sum
  Sum - 5 : Sum  Commented=on
  Switching Frequency (from Initialisation file) : Constant  Value=fs
  Thermal model : Subsystem
  Thermal model 2 : Subsystem  Commented=on
  To Workspace : ToWorkspace  VariableName=P_cond_T1  SaveFormat=Structure With Time  SampleTime=-1
  To Workspace1 : ToWorkspace  VariableName=P_sw_T1  SaveFormat=Structure With Time  SampleTime=-1
  To Workspace10 : ToWorkspace  VariableName=T_cD1  SaveFormat=Structure With Time  SampleTime=-1
  To Workspace2 : ToWorkspace  VariableName=T_jT1  SaveFormat=Structure With Time  SampleTime=-1
  To Workspace3 : ToWorkspace  VariableName=T_jD1  SaveFormat=Structure With Time  SampleTime=-1
  To Workspace4 : ToWorkspace  VariableName=P_cond_D1  SaveFormat=Structure With Time  SampleTime=-1
  To Workspace5 : ToWorkspace  VariableName=P_sw_D1  SaveFormat=Structure With Time  SampleTime=-1
  To Workspace6 : ToWorkspace  VariableName=P_netT1  SaveFormat=Structure With Time  SampleTime=-1
  To Workspace7 : ToWorkspace  VariableName=P_netD1  SaveFormat=Structure With Time  SampleTime=-1
  To Workspace8 : ToWorkspace  VariableName=T_h  SaveFormat=Structure With Time  SampleTime=-1
  To Workspace9 : ToWorkspace  VariableName=T_cT1  SaveFormat=Structure With Time  SampleTime=-1
  per leg1 : Gain  Commented=on  Gain=2
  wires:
  D_abc/1 -> Instantaneous Loss Model/1(D_abc)  "Duty Ratio"
  I_abc/1 -> Instantaneous Loss Model/2(I_abc)  "Three Phase Currents"
  V_dc/1 -> Instantaneous Loss Model/3(V_dc)  "DC link Voltage"
  Switching Frequency (from Initialisation file)/1 -> Instantaneous Loss Model/4(fs)
  Instantaneous Loss Model/1(pconT1_Tj) -> Rate Transition2/1, Sum - 1/1
  Instantaneous Loss Model/2(pswT1_Tj) -> Sum - 1/2, Rate Transition3/1
  Thermal model/1(TjT1) -> Rate Transition5/1, [TjT_M]  "Junction Temperature of Switch"
  Instantaneous Loss Model/3(pconD1_Tj) -> Sum - 2/1, Rate Transition11/1
  Instantaneous Loss Model/4(pswD1_Tj) -> Rate Transition10/1, Sum - 2/2
  Thermal model/4(TcD1) -> Rate Transition9/1, [TcD_M]  "Case Temperature of Diode"
  Thermal model/5(P_T1/D1) -> [P_T1D1]  "Heat Sink Temperature"
  [TjT_M] -> Mux3/1
  [TjD_M] -> Mux3/2
  Mux3/1 -> Instantaneous Loss Model/5(Tj_T1D1)
  Sum - 3/1 -> [pT_M2], Thermal model 2/1(ploss_T2)  "Net Power Loss in Switch"
  Instantaneous Loss Model/5(pconT2_Tj) -> Sum - 3/1
  Instantaneous Loss Model/6(pswT2_Tj) -> Sum - 3/2
  Thermal model 2/1(TjT1) -> [TjT_M2]  "Junction Temperature of Switch"
  Instantaneous Loss Model/7(pconD2_Tj) -> Sum - 4/1
  Instantaneous Loss Model/8(pswD2_Tj) -> Sum - 4/2
  Sum - 4/1 -> [pD_M2], Thermal model 2/2(ploss_D1)  "Net Power Loss in Diode"
  Thermal model 2/2(TjD1) -> [TjD_M2]  "Junction Temperature of Diode"
  Thermal model 2/3(TcT1) -> [TcT_M2]  "Case Temperature of Switch"
  Thermal model 2/4(TcD1) -> [TcD_M2]  "Case Temperature of Diode"
  Thermal model 2/5(TcT2) -> [P_T2D2]  "Power to Heat Sink"
  [TjT_M2] -> Mux1/1
  [TjD_M2] -> Mux1/2
  Mux1/1 -> Instantaneous Loss Model/6(Tj_T2D2)
  Ambient Temperature (from Initialisation file)/1 -> Sum - 5/2
  Sum - 5/1 -> Rate Transition7/1, [Th_gridConv]  "Heat Sink Temperature"
  Heat Sink Model2/1(Tha) -> Sum - 5/1
  Mux/1 -> Scope2/1
  Sum - 1/1 -> [pT_M], Rate Transition1/1, Thermal model/1(ploss_T1)  "Switch Losses"
  Sum - 2/1 -> Thermal model/2(ploss_D1), Rate Transition4/1, [pD_M]  "Diode Losses"
  Thermal model/2(TjD1) -> Rate Transition6/1, [TjD_M]  "Junction Temperature of Switch"
  Rate Transition2/1 -> To Workspace/1
  Rate Transition3/1 -> To Workspace1/1
  Rate Transition1/1 -> Scope4/1, Integrator/1
  Rate Transition4/1 -> Integrator1/1
  Rate Transition5/1 -> Mux/1, To Workspace2/1
  Rate Transition6/1 -> Mux/2, To Workspace3/1
  Rate Transition7/1 -> Scope1/1, To Workspace8/1
  Thermal model/3(TcT1) -> Rate Transition8/1, [TcT_M]  "Junction Temperature of Switch"
  Rate Transition8/1 -> To Workspace9/1
  Rate Transition9/1 -> To Workspace10/1
  Rate Transition10/1 -> To Workspace5/1
  Rate Transition11/1 -> To Workspace4/1
  Integrator/1 -> Scope3/1, To Workspace6/1
  Integrator1/1 -> To Workspace7/1
  per leg1/1 -> Heat Sink Model2/1(PT1/D1)
  [P_T2D2] -> Sum/2
  [P_T1D1] -> per leg1/1
  Ambient Temperature (from Initialisation file)1/1 -> [Th_gridConv]

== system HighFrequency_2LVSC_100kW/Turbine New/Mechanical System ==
  Electric Torque : Inport
  Load Torque : Inport  Port=2
  Gain - 1/J : Gain  Gain=1/J
  Integrator - 1 : Integrator  InitialCondition=omega_m_init
  Sum - 1 : Sum  Inputs=+-  InputSameDT=on  SaturateOnIntegerOverflow=on
  omega_m : Outport  VectorParamsAs1DForOutWhenUnconnected=off
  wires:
  Sum - 1/1 -> Gain - 1/J/1
  Gain - 1/J/1 -> Integrator - 1/1
  Electric Torque/1 -> Sum - 1/1
  Integrator - 1/1 -> omega_m/1  "Generator Rotational Speed"
  Load Torque/1 -> Sum - 1/2

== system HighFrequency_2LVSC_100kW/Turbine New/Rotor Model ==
  note: Power Coefficient
  omega_m : Inport
  Wind Speed : Inport  Port=2
  Cp-lambda : Subsystem
  Divide : Product  Inputs=*/
  Divide1 : Product  Inputs=/*
  Function - Square : Fcn  Expr=u(1)^3
  Gain - 1 : Gain  Gain=-(0.5*rho*A)
  Gain - 2 : Gain
  Gain - 3 : Gain  Gain=Radius
  Product - 1 : Product  RndMeth=Zero
  Scope : Scope
  w_try : Constant  Commented=on  Value=2.4347
  T_load : Outport  VectorParamsAs1DForOutWhenUnconnected=off
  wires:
  Wind Speed/1 -> Divide1/1, Function - Square/1
  Function - Square/1 -> Product - 1/1
  Gain - 1/1 -> T_load/1  "Load Torque"
  Gain - 2/1 -> Product - 1/2
  omega_m/1 -> Gain - 3/1, Divide/2
  Product - 1/1 -> Divide/1
  Divide/1 -> Gain - 1/1
  Gain - 3/1 -> Divide1/2
  Cp-lambda/1(Cp) -> Scope/1, Gain - 2/1
  Divide1/1 -> Cp-lambda/1(lambda)

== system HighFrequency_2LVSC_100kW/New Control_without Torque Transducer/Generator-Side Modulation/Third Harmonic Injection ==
  V_in : Inport
  Gain - 1 : Gain  Gain=1/2
  Max Value : MinMax  Function=max
  Min Value : MinMax
  Sum : Sum  Inputs=|++
  Sum1 : Sum  Inputs=|-+
  V_out : Outport  VectorParamsAs1DForOutWhenUnconnected=off
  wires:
  Sum1/1 -> V_out/1
  Gain - 1/1 -> Sum1/1
  Sum/1 -> Gain - 1/1
  Max Value/1 -> Sum/2
  Min Value/1 -> Sum/1
  V_in/1 -> Sum1/2, Max Value/1, Min Value/1

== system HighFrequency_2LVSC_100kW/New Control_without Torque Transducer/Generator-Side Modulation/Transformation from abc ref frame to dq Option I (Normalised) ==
  D_abc : Inport
  theta_(s) : Inport  Port=2
  Clarke Transform : Subsystem
  Demux : Demux  Outputs=3
  Mux1 : Mux  Inputs=2
  Parks Transform : Subsystem
  D_dq : Outport  VectorParamsAs1DForOutWhenUnconnected=off
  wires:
  Parks Transform/1(out_1) -> Mux1/1
  Parks Transform/2(out_2) -> Mux1/2
  D_abc/1 -> Demux/1
  Mux1/1 -> D_dq/1
  Demux/1 -> Clarke Transform/1(in_1)
  Demux/2 -> Clarke Transform/2(in_2)
  Demux/3 -> Clarke Transform/3(in_3)
  Clarke Transform/1(out_1) -> Parks Transform/1(in_1)
  Clarke Transform/2(out_2) -> Parks Transform/2(in_2)
  theta_(s)/1 -> Parks Transform/3(in_3)

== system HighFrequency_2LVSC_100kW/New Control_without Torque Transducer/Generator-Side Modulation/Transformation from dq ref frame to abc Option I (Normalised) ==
  D_dq : Inport
  theta : Inport  Port=2
  Clarke Transform : Subsystem
  Demux : Demux  Outputs=2
  Gain : Gain  Gain=-1
  Mux1 : Mux  Inputs=3
  Parks Transform : Subsystem
  D_abc : Outport  VectorParamsAs1DForOutWhenUnconnected=off
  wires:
  Parks Transform/2(out_2) -> Clarke Transform/2(in_2)
  Parks Transform/1(out_1) -> Clarke Transform/1(in_1)
  Gain/1 -> Parks Transform/3(in_3)
  D_dq/1 -> Demux/1
  Mux1/1 -> D_abc/1
  Demux/1 -> Parks Transform/1(in_1)
  Demux/2 -> Parks Transform/2(in_2)
  theta/1 -> Gain/1
  Clarke Transform/3(out_3) -> Mux1/3
  Clarke Transform/2(out_2) -> Mux1/2
  Clarke Transform/1(out_1) -> Mux1/1

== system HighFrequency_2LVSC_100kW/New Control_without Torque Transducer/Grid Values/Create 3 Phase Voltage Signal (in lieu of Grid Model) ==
  Grid Voltage : Inport
  Phase - A : Sin  Amplitude=sqrt(2)  Frequency=omega_s  Phase=Usfi0
  Phase - B : Sin  Amplitude=sqrt(2)  Frequency=omega_s  Phase=-2*pi/3+Usfi0
  Phase - C : Sin  Amplitude=sqrt(2)  Frequency=omega_s  Phase=-4*pi/3+Usfi0
  Product - 1 : Product  InputSameDT=on  RndMeth=Zero  SaturateOnIntegerOverflow=on
  Product - 2 : Product  InputSameDT=on  RndMeth=Zero  SaturateOnIntegerOverflow=on
  Product - 3 : Product  InputSameDT=on  RndMeth=Zero  SaturateOnIntegerOverflow=on
  Phase A Voltage : Outport  VectorParamsAs1DForOutWhenUnconnected=off
  Phase B Voltage : Outport  Port=2  VectorParamsAs1DForOutWhenUnconnected=off
  Phase C Voltage : Outport  Port=3  VectorParamsAs1DForOutWhenUnconnected=off
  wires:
  Grid Voltage/1 -> Product - 3/2, Product - 1/2, Product - 2/2
  Phase - C/1 -> Product - 3/1
  Phase - B/1 -> Product - 2/1
  Phase - A/1 -> Product - 1/1
  Product - 1/1 -> Phase A Voltage/1
  Product - 2/1 -> Phase B Voltage/1
  Product - 3/1 -> Phase C Voltage/1

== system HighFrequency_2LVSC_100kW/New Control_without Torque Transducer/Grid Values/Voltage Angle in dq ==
  Three Phase Voltages : Inport
  Demux : Demux  Outputs=3
  Normalized Clarke Transform : Subsystem
  S Function : MATLAB Function  TreatAsAtomicUnit=on
  Terminator - 1 : Terminator
  angle : Outport  VectorParamsAs1DForOutWhenUnconnected=off
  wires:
  Demux/3 -> Normalized Clarke Transform/3(c)
  Demux/1 -> Normalized Clarke Transform/1(a)
  Demux/2 -> Normalized Clarke Transform/2(b)
  Three Phase Voltages/1 -> Demux/1
  S Function/1(angle) -> angle/1
  Normalized Clarke Transform/1(alpha) -> S Function/1(x)
  Normalized Clarke Transform/2(beta) -> S Function/2(y)
  Normalized Clarke Transform/3(zero) -> Terminator - 1/1  "Zero Sequence is 0 for balanced systems"

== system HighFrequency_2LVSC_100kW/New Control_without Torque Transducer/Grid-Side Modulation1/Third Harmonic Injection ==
  V_in : Inport
  Gain - 1 : Gain  Gain=1/2
  Max Value : MinMax  Function=max
  Min Value : MinMax
  Sum : Sum  Inputs=|++
  Sum1 : Sum  Inputs=|-+
  V_out : Outport  VectorParamsAs1DForOutWhenUnconnected=off
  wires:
  Sum1/1 -> V_out/1
  Gain - 1/1 -> Sum1/1
  Sum/1 -> Gain - 1/1
  Max Value/1 -> Sum/2
  Min Value/1 -> Sum/1
  V_in/1 -> Sum1/2, Max Value/1, Min Value/1

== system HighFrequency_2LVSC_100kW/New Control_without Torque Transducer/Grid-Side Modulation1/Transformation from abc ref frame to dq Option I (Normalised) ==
  D_abc : Inport
  theta_(s) : Inport  Port=2
  Clarke Transform : Subsystem
  Demux : Demux  Outputs=3
  Mux1 : Mux  Inputs=2
  Parks Transform : Subsystem
  D_dq : Outport  VectorParamsAs1DForOutWhenUnconnected=off
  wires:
  Parks Transform/1(out_1) -> Mux1/1
  Parks Transform/2(out_2) -> Mux1/2
  D_abc/1 -> Demux/1
  Mux1/1 -> D_dq/1
  Demux/1 -> Clarke Transform/1(in_1)
  Demux/2 -> Clarke Transform/2(in_2)
  Demux/3 -> Clarke Transform/3(in_3)
  Clarke Transform/1(out_1) -> Parks Transform/1(in_1)
  Clarke Transform/2(out_2) -> Parks Transform/2(in_2)
  theta_(s)/1 -> Parks Transform/3(in_3)

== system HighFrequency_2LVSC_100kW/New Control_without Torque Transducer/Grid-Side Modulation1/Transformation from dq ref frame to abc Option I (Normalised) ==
  D_dq : Inport
  theta : Inport  Port=2
  Clarke Transform : Subsystem
  Demux : Demux  Outputs=2
  Gain : Gain  Gain=-1
  Mux1 : Mux  Inputs=3
  Parks Transform : Subsystem
  D_abc : Outport  VectorParamsAs1DForOutWhenUnconnected=off
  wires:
  Parks Transform/2(out_2) -> Clarke Transform/2(in_2)
  Parks Transform/1(out_1) -> Clarke Transform/1(in_1)
  Gain/1 -> Parks Transform/3(in_3)
  D_dq/1 -> Demux/1
  Mux1/1 -> D_abc/1
  Demux/1 -> Parks Transform/1(in_1)
  Demux/2 -> Parks Transform/2(in_2)
  theta/1 -> Gain/1
  Clarke Transform/3(out_3) -> Mux1/3
  Clarke Transform/2(out_2) -> Mux1/2
  Clarke Transform/1(out_1) -> Mux1/1

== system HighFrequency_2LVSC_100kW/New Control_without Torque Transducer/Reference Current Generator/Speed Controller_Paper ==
  N : Inport
  N* : Inport  Port=2
  Constant4 : Constant  Value=T_overrating
  Constant5 : Constant  Value=-1
  IC : InitialCondition  Value=0
  Low pass filter : DiscreteTransferFcn  Numerator=[1-exp(-2*pi*fc*Tsc)]  Denominator=[1 -exp(-2*pi*fc*Tsc)]  SampleTime=Tsc
  PID Controller : pid_lib/PID Controller  Controller=PI  Form=Parallel  TimeDomain=Discrete-time  UseExternalTs=off  SampleTime=-1  IntegratorMethod=Forward Euler  FilterMethod=Forward Euler  ControllerParametersSource=internal  P=kp  I=ki  D=10  UseFilter=on  N=100  TunerSelectOption=Transfer Function Based (PID Tuner App)  InitialConditionSource=internal  InitialConditionForIntegrator=0  InitialConditionForFilter=0  DifferentiatorICPrevScaledInput=0  ExternalReset=none  TrackingMode=off  Kt=1  LimitOutput=on  SatLimitsSource=internal  UpperSaturationLimit=-1  LowerSaturationLimit=T_overrating  LinearizeAsGain=on  AntiWindupMode=clamping  Kb=1  POutMin=[]  POutMax=[]  IOutMin=[]  IOutMax=[]  DOutMin=[]  DOutMax=[]  NOutMin=[]  NOutMax=[]  SumOutMin=[]  SumOutMax=[]  SaturationOutMin=[]  SaturationOutMax=[]  PParamMin=[]  PParamMax=[]  IParamMin=[]  IParamMax=[]  DParamMin=[]  DParamMax=[]  NParamMin=[]  NParamMax=[]  KbParamMin=[]  KbParamMax=[]  KtParamMin=[]  KtParamMax=[]  KbOutMin=[]  KbOutMax=[]  KtOutMin=[]  KtOutMax=[]  IntegratorOutMin=[]  IntegratorOutMax=[]  FilterOutMin=[]  FilterOutMax=[]  SumI1OutMin=[]  SumI1OutMax=[]  SumI2OutMin=[]  SumI2OutMax=[]  SumI3OutMin=[]  SumI3OutMax=[]  SumI4OutMin=[]  SumI4OutMax=[]  SumDOutMin=[]  SumDOutMax=[]  DifferentiatorOutMin=[]  DifferentiatorOutMax=[]  FilterDiffOutCoefMin=[]  FilterDiffOutCoefMax=[]  ReciprocalOutMin=[]  ReciprocalOutMax=[]  SumDenOutMin=[]  SumDenOutMax=[]  SumNumOutMin=[]  SumNumOutMax=[]  DivideOutMin=[]  DivideOutMax=[]  UdiffTsProdOutMin=[]  UdiffTsProdOutMax=[]  NTsProdOutMin=[]  NTsProdOutMax=[]  UintegralTsProdOutMin=[]  UintegralTsProdOutMax=[]  UngainTsProdOutMin=[]  UngainTsProdOutMax=[]  IntegratorContinuousStateAttributes=''  IntegratorStateMustResolveToSignalObject=off  IntegratorRTWStateStorageClass=Auto  FilterContinuousStateAttributes=''  FilterStateMustResolveToSignalObject=off  FilterRTWStateStorageClass=Auto  ParallelPVariant=InternalParameters  IdealPVariant=Disabled  IVariant=InternalParameters  DVariant=Disabled  IntegratorVariant=Discrete  SatVariant=Enabled  AWVariant=DiscClampingParallel  PCopyVariant=Disabled  TRVariant=Disabled  FdbkBlocksVariant=Forward  IdealPFdbkVariant=Disabled  SatFdbkVariant=Disabled  DerivativeFilterVariant=Disabled  NVariant=Disabled  NCopyVariant=Disabled_SignalSpec  FilterICVariant=Disabled  IntegratorICVariant=InternalICs  ExternalResetVariant=Disabled  TRSumVariant=Passthrough  SumFdbkVariant=Disabled  SumVariant=Sum_PI  TsampFilterVariant=InternalTs  TsampNgainVariant=Passthrough  TsampIntegralVariant=Passthrough  ExternalSaturationOutDataTypeStr=Inherit: Same as second input
  Rate Limiter : RateLimiter  RisingSlewLimit=ramp(2)  FallingSlewLimit=ramp(1)  LinearizeAsGain=off
  Rate Transition : RateTransition
  Saturation Dynamic : simulink/Discontinuities/Saturation Dynamic  OutMin=[]  OutMax=[]  OutDataTypeStr=Inherit: Same as second input  OutDataType=fixdt(1, 16)  OutScaling=2^-10  DoSatur=off
  Sum1 : Sum  Inputs=|+-  InputSameDT=on  SaturateOnIntegerOverflow=on
  Zero-Order Hold1 : ZeroOrderHold  SampleTime=Tsc
  Zero-Order Hold5 : ZeroOrderHold  SampleTime=Tsc
  Torque* : Outport  VectorParamsAs1DForOutWhenUnconnected=off
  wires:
  Zero-Order Hold5/1 -> Sum1/1
  N*/1 -> IC/1
  Low pass filter/1 -> Sum1/2
  Zero-Order Hold1/1 -> Low pass filter/1
  IC/1 -> Rate Limiter/1
  Rate Transition/1 -> Torque*/1
  N/1 -> Zero-Order Hold1/1
  Saturation Dynamic/1 -> Rate Transition/1  "Torque reference (Nm)"
  Sum1/1 -> PID Controller/1  "Error"
  Rate Limiter/1 -> Zero-Order Hold5/1
  PID Controller/1 -> Saturation Dynamic/2
  Constant5/1 -> Saturation Dynamic/1
  Constant4/1 -> Saturation Dynamic/3
